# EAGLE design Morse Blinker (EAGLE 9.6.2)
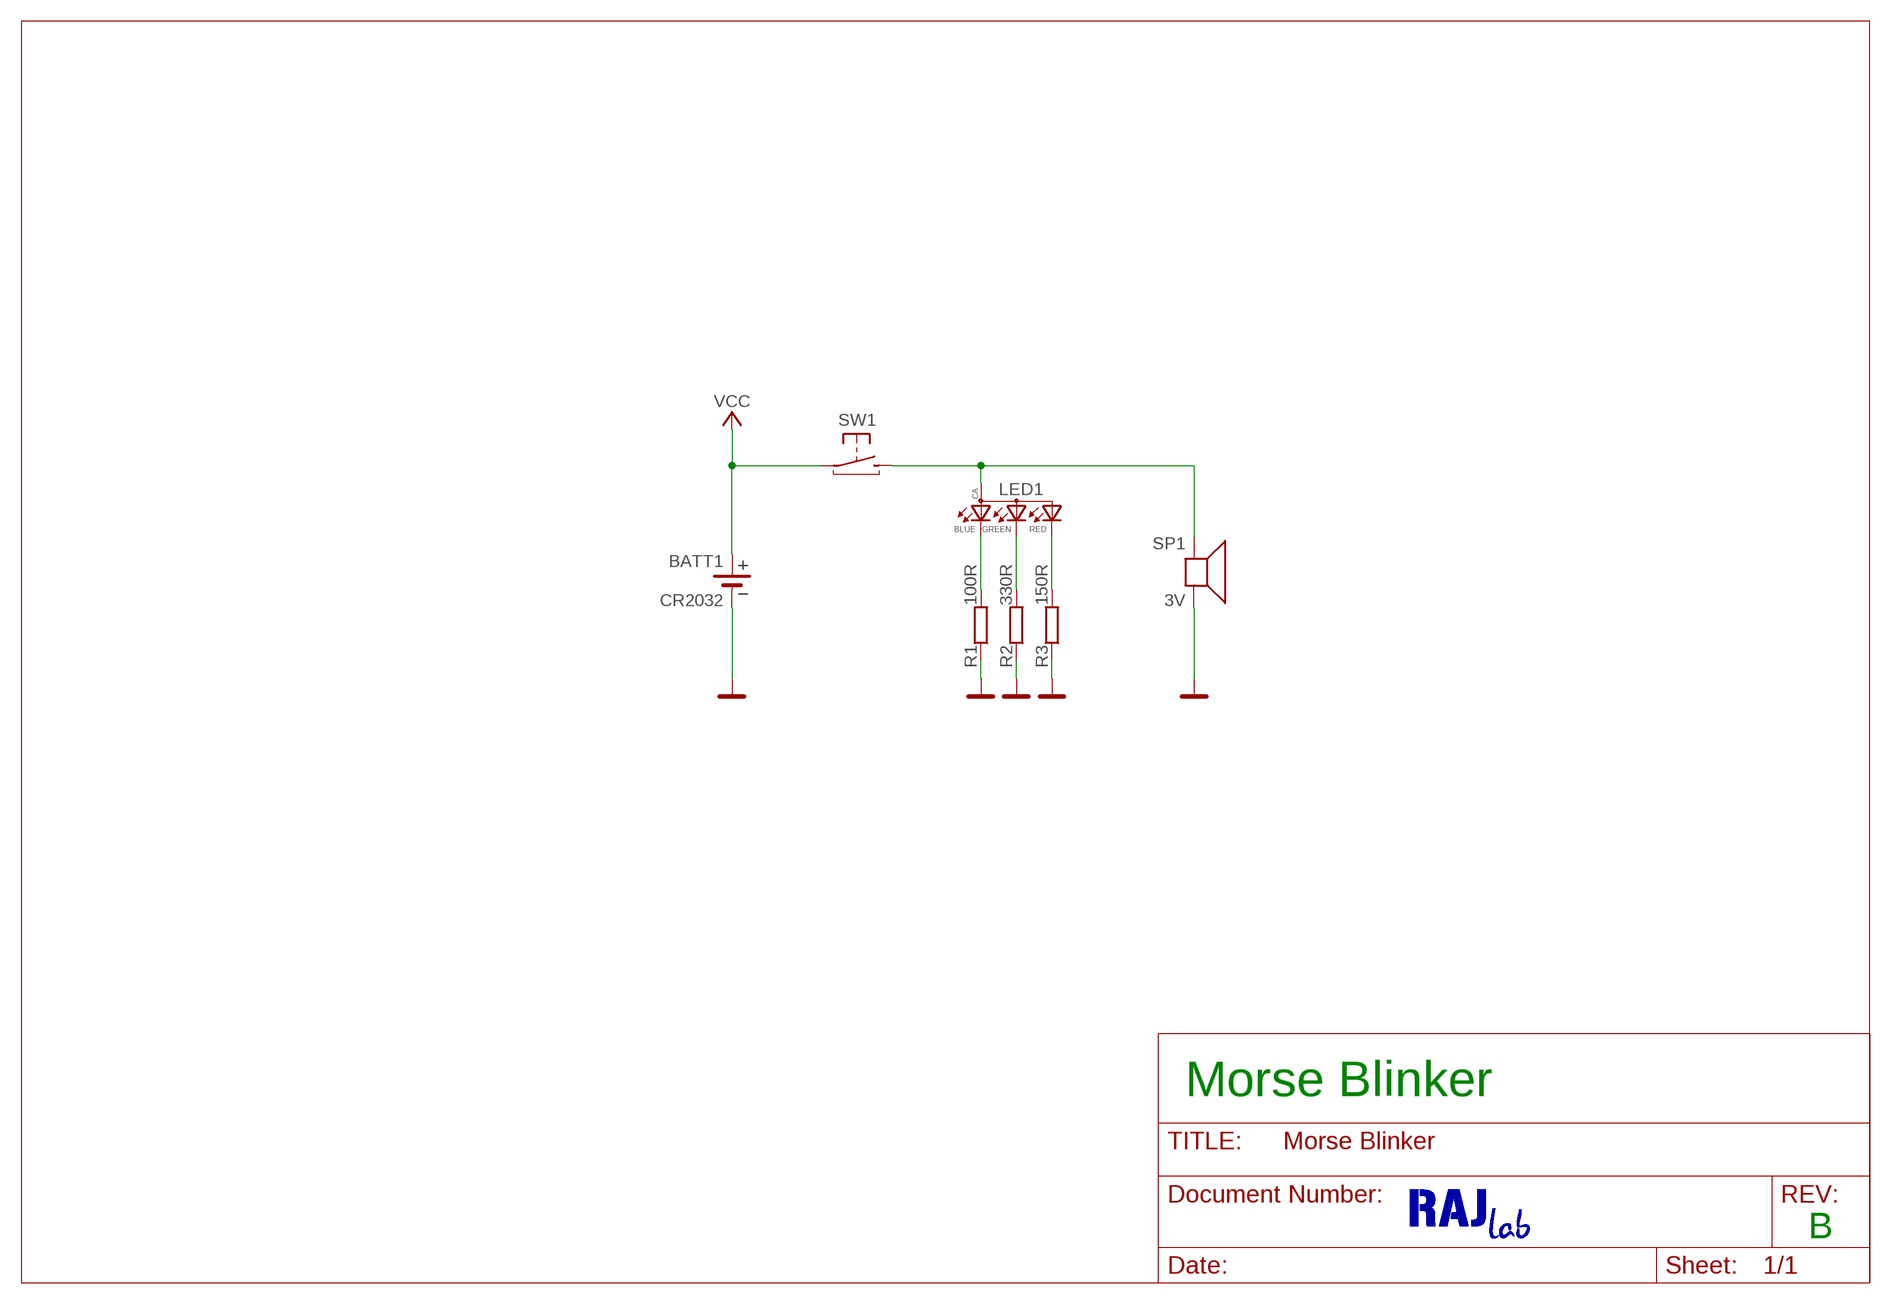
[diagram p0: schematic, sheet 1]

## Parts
BATT1  CR2032  MY-2032-12  [CR2032_SMT]
LED1  RF-W2SA30BS-A15(WE)  [3528/PLCC4_BLACK]
R1  100R  R-EU_R0805  [R0805]
R2  330R  R-EU_R0805  [R0805]
R3  150R  R-EU_R0805  [R0805]
SP1  3V  BUZZER_12095  [12095]
SW1  GENERIC_6X6X4.5  [TACT-SW_6X6X4.5_SMT]

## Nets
GND: BATT1.- R1.1 R2.1 R3.1 SP1.-
N$2: LED1.2(ANODE) SP1.+ SW1.S1(S) SW1.S2(S)
N$3: LED1.1(BLUE) R1.2
N$4: LED1.4(GREEN) R2.2
N$5: LED1.3(RED) R3.2
VCC: BATT1.+1(+) BATT1.+2(+) SW1.P1(P) SW1.P2(P)

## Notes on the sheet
- Morse Blinker
- B

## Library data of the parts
BATT1 = #oktkas-battery:MY-2032-12: CR2032 / LIR2032 SMT battery holder; LCSC_PART: C964833
LED1 = #oktkas-led:RF-W2SA30BS-A15(WE): Cheap RGB LED | TME link
R1-R3 = rcl:R-EU_: RESISTOR, European symbol; SPICEPREFIX: R
SP1 = #oktkas-speaker:BUZZER
SW1 = #oktkas-buttons:GENERIC: Generic tactile buttons and footprint combinations; LCSC_PART: C127509

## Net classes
0 default: width 0.127 mm, drill 0.2 mm, clearance 0.127 mm

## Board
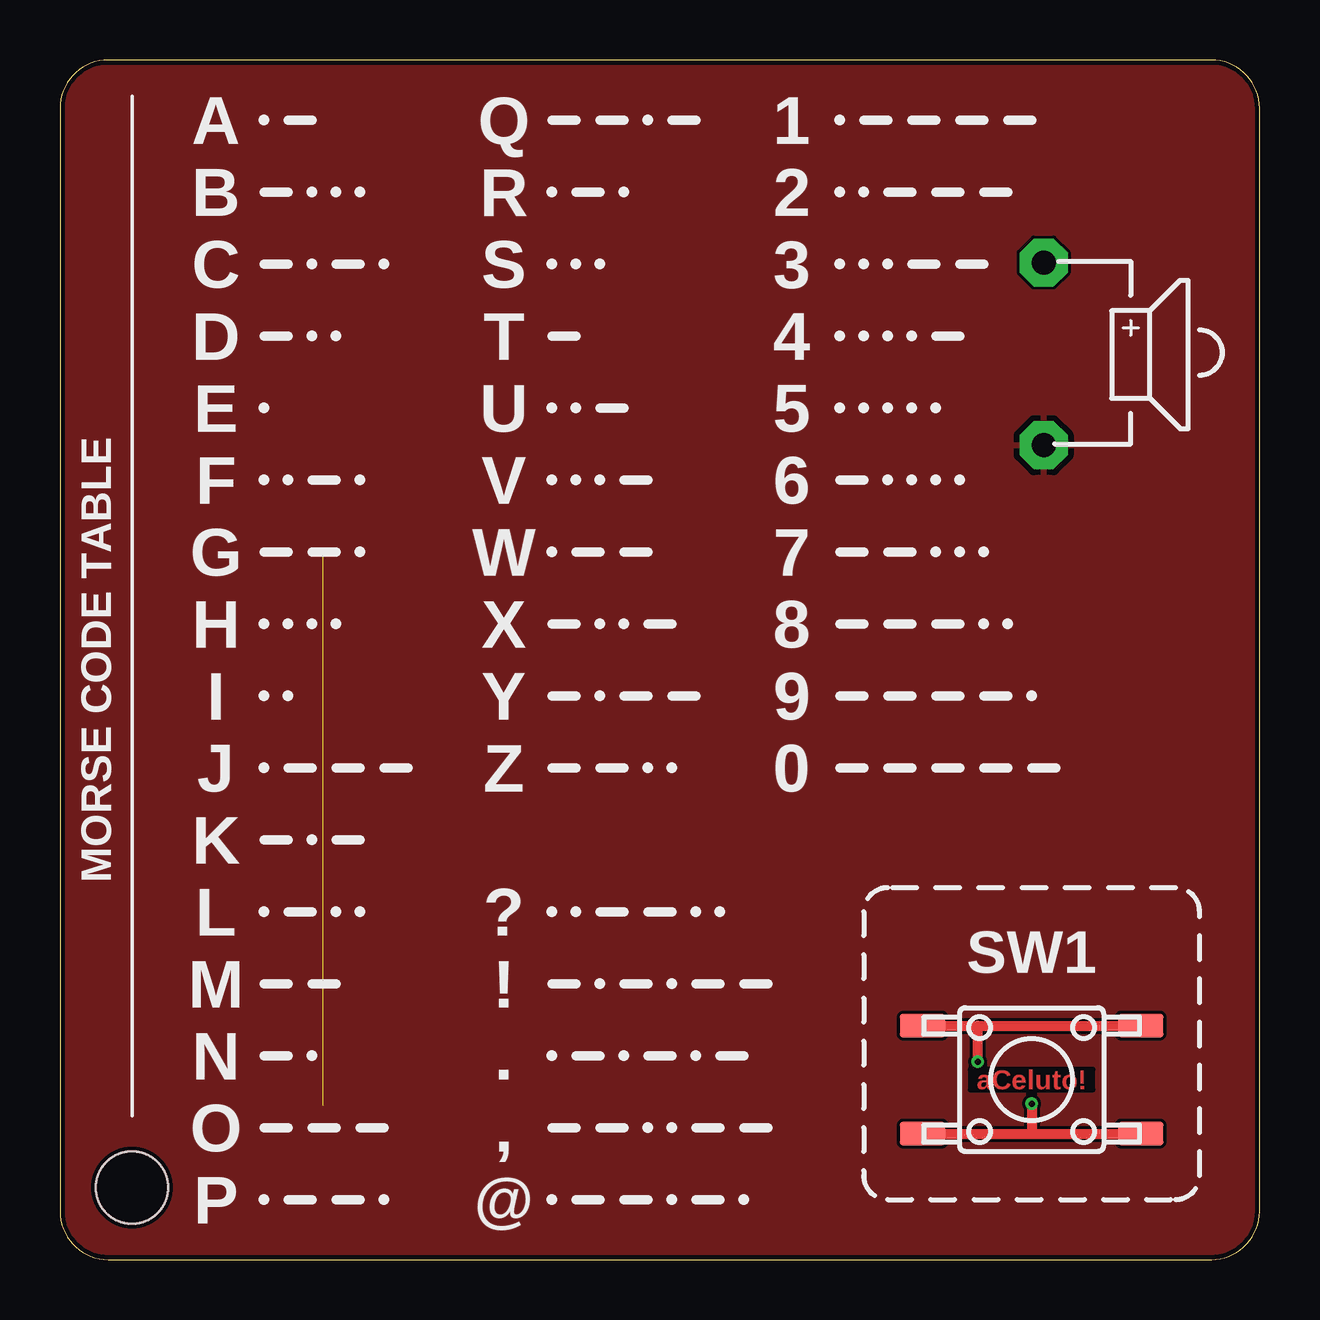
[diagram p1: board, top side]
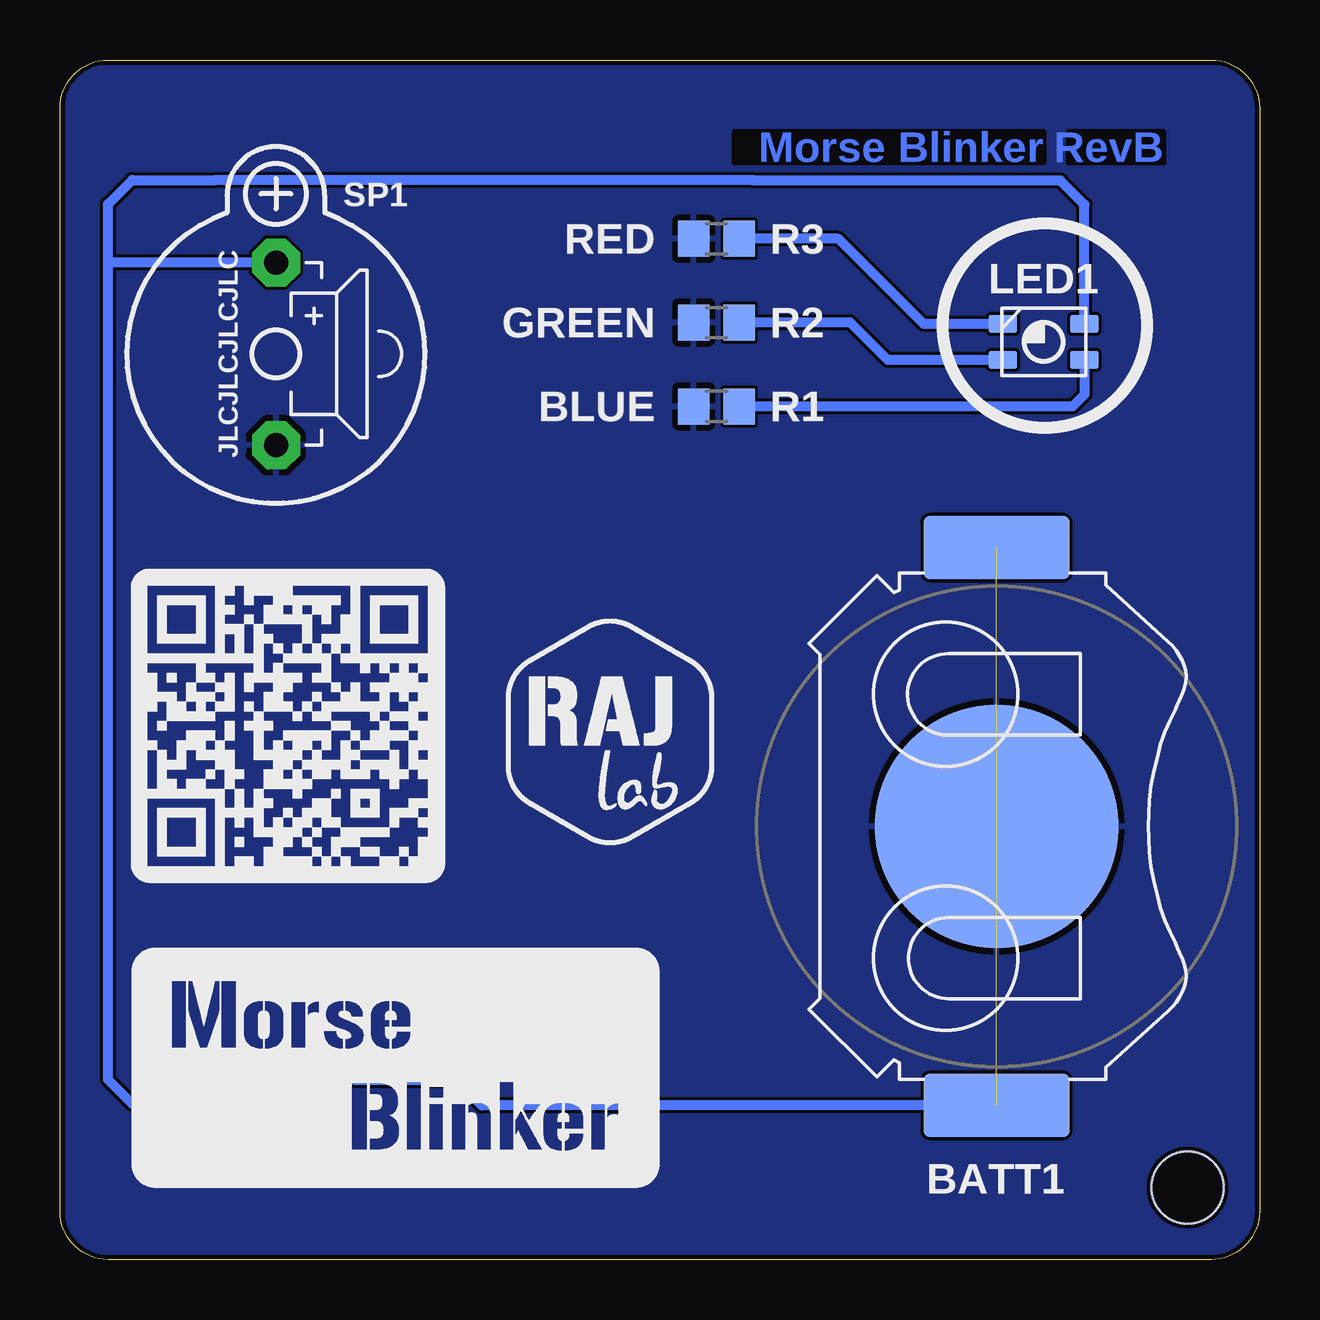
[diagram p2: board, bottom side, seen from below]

Size 50 x 50 mm. Coordinates in mm from the lower left corner, seen from the top.
Outline: 48,50 2,50 arc90 0,48 0,2 arc90 2,0 48,0 arc90 50,2 50,48 arc90 48,50
Copper layers (1*16): Top 0.035mm / dielectric 1.6mm / Bottom 0.035mm
Design rules "jlcpcb-2layers_od-Ondry3-assembly-tight": minimum track width 5mil, minimum drill 0.2mm, track to track 5mil, track to pad 5mil, pad to pad 5mil, via to via 5mil, smd to smd 5mil, copper to edge 0.2mm, drill to drill 6mil, minimum pad ring 0.13mm, minimum via ring 0.13mm, stop-mask expansion 4mil, vias tented up to drill 0.6mm, thermal gap 10mil
Holes 3 mm at 3,3

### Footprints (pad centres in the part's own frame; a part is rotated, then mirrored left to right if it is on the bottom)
CR2032_SMT = smd 2.65 x 6.1: +1 -11.625,0; +2 11.625,0 | smd 10.16 x 10.16: - 0,0
3528/PLCC4_BLACK = smd 1.2 x 0.75: 1 1.7,-0.75; 2 1.7,0.75; 3 -1.7,0.75; 4 -1.7,-0.75
R0805 = smd 1.3 x 1.5: 1 -0.95,0; 2 0.95,0
12095 = drill 1 pad 2 octagon: + 0,3.81; - 0,-3.81
TACT-SW_6X6X4.5_SMT = smd 1.9 x 1: P1 -4.55,2.25; P2 4.55,2.25; S1 -4.55,-2.25; S2 4.55,-2.25

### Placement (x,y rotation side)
BATT1  10.96,18.05 90 bottom
LED1  9,38.25 0 bottom
R1  22.64,35.56 0 bottom
R2  22.64,39.05 0 bottom
R3  22.64,42.55 0 bottom
SP1  41,37.75 0 bottom
SW1  40.5,7.5 0 top
U$12  [RAJLAB-HEX_10MM_N]  27,22 0 bottom

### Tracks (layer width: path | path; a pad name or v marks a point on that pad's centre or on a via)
GND
  pour Bottom: 0,48.01 0,2 arc90 2,0 48.01,0 arc90 50.01,2 50.01,48.01 arc90 48.01,50.01 2,50.01 arc90
  pour Top: 48.01,0 2,0 arc-90 0,2 0,48.01 arc-90 2,50.01 48.01,50.01 arc-90 50.01,48.01 50.01,2 arc-90
N$2  (via drill 0.25)
  Top 0.406: SW1.S1 40.5,5.25 | 40.5,5.25 SW1.S2 | v40.5,6.5 40.5,5.25
  Bottom 0.406: v40.5,6.5 43.5,6.5 47,6.5 48,7.5 48,41.5 | LED1.2 7.3,43.98 8.3,44.98 21.11,44.98 21.13,45 43.5,45 47,45 48,44 48,41.5 | SP1.+ 43.94,41.56 47.94,41.56 48,41.5
N$3
  Bottom 0.406: LED1.1 7.3,36.06 7.8,35.56 R1.2
N$4
  Bottom 0.406: LED1.4 15.5,37.5 17.05,39.05 R2.2
N$5
  Bottom 0.406: LED1.3 14,39 17.55,42.55 R3.2
VCC  (via drill 0.25)  (1 unrouted)
  Top 0.406: SW1.P1 38.25,9.75 | 38.25,9.75 SW1.P2 | v38.25,8.25 38.25,9.75
  Bottom 0.406: BATT1.+1 32.42,6.42 33.5,7.5 37.75,7.5 38.25,8 v38.25,8.25

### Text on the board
Top: aCeluto!
Bottom: RevB
tPlace: A | Q | 1 | B | R | 2 | C | S | 3 | D | T | 4 | E | U | 5 | F | V | 6 | G | W | 7 | H | X | 8 | MORSE CODE TABLE | I | Y | 9 | J | Z | 0 | K | L | ? | M | ! | N | . | O | , | P | @
bPlace: JLCJLCJLCJLC
bNames: RED | GREEN | BLUE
